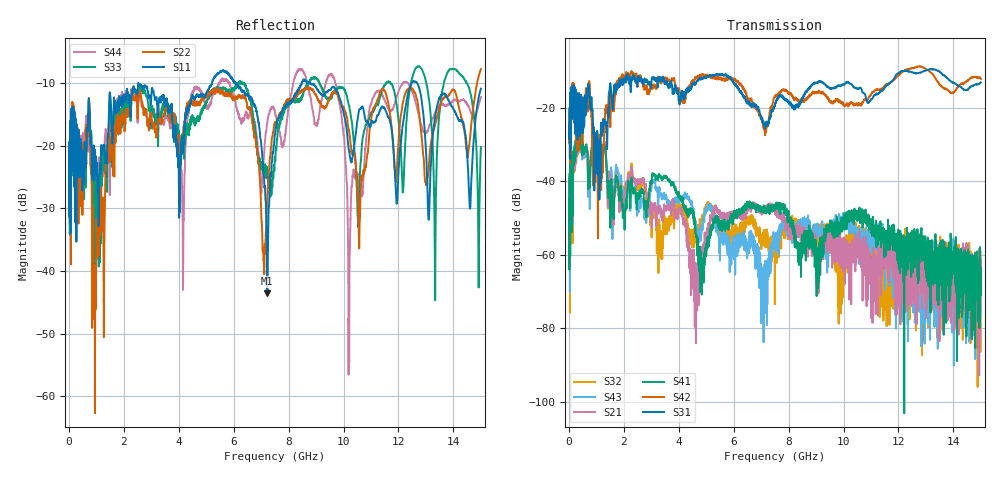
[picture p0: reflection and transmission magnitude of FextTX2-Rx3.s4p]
! FILE: N:\QM 2007\Prüfprotokolle\Highspeed\Konfektionierte Ltg\L45593-D106\D30\8216\0002\Fext\FextTX2-Rx3.s4p
# MHz S MA R 50.00
! FREQ  S11  S12  S13  S14
!  S21  S22  S23  S24
!  S31  S32  S33  S34
!  S41  S42  S43  S44
!  MAG  ANG  MAG  ANG  MAG  ANG  MAG  ANG
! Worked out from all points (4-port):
!   2999 points, 10 MHz to 15 GHz, reference 50 ohm
!   strongest paths, dB at 10 MHz, 3.755 GHz, 7.505 GHz, 11.26 GHz, 15 GHz:
!     S31: -26.1, -13.6, -19.2, -16.1, -13.1
!     S42: -24.3, -11.9, -17.1, -15.1, -12.1
!     S41: -44.9, -40.7, -47.5, -53.2, -65.1
!     S21: -51.0, -45.9, -48.6, -76.4, -63.3
!     S43: -43.3, -45.9, -54.5, -52.2, -67.6
!     S32: -45.9, -48.1, -59.1, -67.6, -62.2
!   lowest |S11| = -43.5 dB at 7.225 GHz (marker M1), VSWR 1.01, Z = 50.4 + j0.514 ohm
!   |S11| at or under -10 dB: start of sweep to 5.214 GHz; 6.071 GHz to 8.48 GHz (2.409 GHz wide, 33.1 % of centre); 8.78 GHz to 12.49 GHz (3.709 GHz wide, 34.9 % of centre)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
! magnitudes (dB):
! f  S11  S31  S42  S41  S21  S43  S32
! 10 MHz  -19.5  -26.1  -24.3  -44.9  -51.0  -43.3  -45.9
! 1.28 GHz  -20.4  -23.9  -27.5  -30.4  -29.4  -29.8  -29.2
! 4.645 GHz  -11.8  -13.0  -11.9  -54.6  -69.8  -51.8  -53.2
! 7.225 GHz  -43.5  -23.8  -24.6  -48.1  -46.6  -73.4  -53.8
! 9.61 GHz  -10.6  -14.6  -18.3  -53.0  -58.4  -55.7  -55.5
! 10.21 GHz  -21.2  -13.2  -18.9  -49.9  -61.5  -50.7  -54.0
! 15 GHz  -10.9  -13.1  -12.1  -65.1  -63.3  -67.6  -62.2
